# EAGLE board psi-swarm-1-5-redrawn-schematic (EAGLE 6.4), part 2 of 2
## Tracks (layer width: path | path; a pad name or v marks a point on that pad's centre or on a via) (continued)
N$38  (via drill 0.25 pad 0.65, 0.35 pad 0.75) (continued)
  Top 0.3: v24.6,17.68 23.1,17.68 22.55,18.23 22.55,20.08 22.45,20.18
  Top 0.305: U$16.P$2 79.9,19.58 78,17.68 76.6,17.68 73.7,14.78 62.3,14.78 v62.2,14.68 | 22.45,20.18 22.45,21.63 21.9,22.18 19.6,22.18 v19.5,22.28 | v15.05,22.38 U$17.3
  Bottom 0.305: v62.2,14.68 62.2,11.58 61.2,10.58 57.5,10.58 55.6,8.68 46.7,8.68 45,10.28 42.05,10.28 41.45,9.68 36.1,9.68 35.5,10.28 34.95,10.78 35,16.28 34.4,16.88 28.9,16.88 27.7,18.08 24.7,18.08 24.6,17.98 v24.6,17.68 | v19.5,22.28 15.15,22.28 v15.05,22.38
N$39  (via drill 0.25 pad 0.6)
  Top 0.2: IR3.CATHODE 99.46,32.29 98.97,32.78 | 98.97,32.78 N2.3 | v97.5,28.28 96.8,28.28 96.8,32.78 98.97,32.78 | v32,6.98 33,7.88 37.8,6.18 36.6,3.58 39.6,2.58 46.4,1.28 48,1.58 v48,1.88
  Top 0.254: IR5.CATHODE 30.7,7.28 v31.7,9.88 | v11.1,24.28 11,24.28 11,24.78 8,24.78 5.1,29.48 7.1,30.38 7.1,30.58 5.6,33.88 5.2,33.98 3.1,33.18 IR6.CATHODE
  Bottom 0.2: IR4.CATHODE 70.49,5.78 69.7,6.58 | 69.7,6.58 69.5,7.08 | 74.6,9.08 75.5,6.68 80.2,9.18 85.8,13.38 91.3,19.18 v97.5,28.28 | IR5.CATHODE 31.3,5.38 v32,6.98 | v48,1.88 48,1.58 55.7,1.58 61.8,2.48 67.9,4.18 67.4,5.58 69.7,6.58
  Bottom 0.254: v31.7,9.88 31.6,9.68 27.7,11.38 27.2,11.18 27.1,11.08 26.4,9.78 22.8,11.78 19.5,14.58 18.95,15.13 18.95,15.78 18.45,16.28 17.5,16.28 14.3,19.48 14.3,20.28 13.9,20.78 13.2,20.78 12.9,20.38 11,22.38 11,24.18 v11.1,24.28 | 74.6,9.08 73.8,8.78 73.6,9.28 73.1,9.48 72.4,9.18 72.2,8.38 69.5,7.08
N$40  (via drill 0.25 pad 0.6)
  Top 0.254: v54.7,98.88 RA3.1A
  Bottom 0.2: 31.8,99.08 33.2,99.08 33.9,99.78 37,100.88 37.5,100.88 38.1,101.08
  Bottom 0.25: 38.1,101.08 38.1,101.58 38.5,101.98
  Bottom 0.254: 27.8,98.88 27.8,99.06 IR_B1.P1-ANODE 29.3,98.78 31.3,99.58 31.8,99.08 | 38.5,101.98 41.9,102.78 41.9,103.18 43.2,103.48 44.5,102.18 49.7,102.18 52.3,99.58 54.7,99.58 v54.7,98.88
N$41  (via drill 0.25 pad 0.65)
  Top 0.2: U$15.3 19.66,28.23 U$15.8 | v28.7,66.48 31.2,68.98 34.5,68.98 v34.8,69.28 | v34.8,84.18 34.8,85.63 R26.2 | 22.25,29.78 22.25,28.3 U$4.10
  Top 0.254: C1.1 22.1,30.28 22,30.18 | 20.43,28.28 U$15.3
  Top 0.305: 22.14,28.04 22,28.18
  Top 0.6: 20.43,28.28 20.43,28.3 20.55,28.43 21.75,28.43 | 21.75,28.43 22,28.18 | 22,30.18 22,28.68 21.75,28.43 | 22.14,28.04 22.14,29.67 22.25,29.78
  Top 0.61: U$2.+ 22.95,39.71 22.95,31.73 22.6,31.38 C1.1
  Bottom 0.2: U$2.+ 24.04,43.44 21.2,46.28 21.2,47.08 21,47.28 21,47.98 21.4,48.38 21.4,55.68 25.8,60.08 27.6,60.08 28.8,61.28 28.8,66.38 v28.7,66.48 | v34.8,69.28 v34.8,84.18
N$42
  Top 0.2: U$4.9 22.99,29.07 23,29.08 23.5,29.08 23.7,29.28 23.7,36.78 25.6,38.68 29.3,38.68 30.2,37.68 35.65,37.68 TH1.2
N$43
  Top 0.61: HB_L.P$1 37.7,55.48 32.1,55.48 32.1,58.48 LEFT_MOTOR.MOTOR+
N$44
  Top 0.61: LEFT_MOTOR.MOTOR- 32,53.18 36.4,53.18 36.4,51.22 HB_L.P$7
N$46  (via drill 0.25 pad 0.6)
  Top 0.254: v49.1,100.28 49,100.18 47.74,100.18 RA1.3A
  Bottom 0.254: IR1.ANODE 72.6,100.38 58.6,100.38 57.9,99.68 55.9,99.68 55.5,99.28 55.5,98.68 55.1,98.18 51.3,98.18 v49.1,100.28
N$47  (via drill 0.25 pad 0.6)
  Top 0.2: RA1.4A 47.1,98.28 47.1,97.18 47.3,96.98 v47.8,96.98
  Top 0.254: v96.15,78.53 96.3,78.38 99,71.58 IR2.ANODE
  Bottom 0.2: 88.1,89.28 88.1,87.68 87.55,87.13 87.55,86.63 87.8,86.33 88.75,86.33 90.1,87.68 94.14,82.87 | v47.8,96.98 49,96.98 49.5,96.48 54,96.48 55.8,94.68 59.8,94.68 60.9,95.78 61.1,95.78
  Bottom 0.254: 61.1,95.78 81.5,95.78 81.6,95.68 83.9,93.53 84.55,93.53 85.4,92.78 85.4,91.98 88.1,89.28 | 93.9,83.18 94.14,82.87 95,81.78 96.4,78.93 v96.15,78.53
N$48  (via drill 0.25 pad 0.6, 0.25 pad 0.65)
  Top 0.2: v67.6,31.78 67.4,31.98 55.4,31.98 55,32.38 34.4,32.38 v34.1,32.08 | v11.9,29.38 RA2.1A
  Bottom 0.2: IR3.ANODE 92.87,31.11 92.45,31.58 91.5,31.58 90.4,30.48 89.6,30.48 88.85,31.13 82.85,31.13 82.2,31.78 80.95,31.78 80.5,31.38 73.2,31.38 72.8,30.98 71.5,30.98 71.1,31.38 68,31.38 v67.6,31.78 | v34.1,32.08 20.6,32.08 19.55,33.13 17.6,33.13 16.55,32.78 16.25,32.48 16.25,30.38 12,30.38 RA2.1A v11.9,29.38
N$49  (via drill 0.25 pad 0.65)
  Top 0.2: v13.15,29.38 13.15,30.26 RA2.2A
  Bottom 0.2: IR4.ANODE 68.94,4.42 68.1,3.58 62.2,1.98 54.8,0.98 46,1.08 39.3,2.28 34.9,3.68 36,6.48 27.8,10.08 27.7,9.98 26.9,8.18 21.8,11.08 15.9,15.88 10.5,22.08 10.5,24.58 11.8,25.88 11.8,26.48 12.4,27.08 12.85,27.08 13.6,27.83 13.6,28.93 v13.15,29.38
N$50  (via drill 0.25 pad 0.6)
  Top 0.2: RA2.3A 14.45,31.18 9.55,31.18 v9.35,30.98
  Bottom 0.254: IR5.ANODE 26.9,6.98 20.9,10.38 14.4,15.58 9.1,21.88 9.1,24.08 9.4,24.38 v9.35,30.98
N$51
  Top 0.2: RA2.4A 15.71,31.42 15.35,31.78 7.25,31.78 7,32.03 6.05,34.38 4.65,34.68 3.9,36.53 IR6.ANODE
N$52  (via drill 0.25 pad 0.6)
  Top 0.2: v9.1,75.38 8.9,75.48 9.6,77.08 9.7,78.18 9.1,79.78 8.9,79.98 10.1,82.08 11.4,82.08 12.1,82.68 12.1,84.18 11.9,84.38 11.9,85.58 12.4,86.28 23.8,86.28 24,86.48 25,86.48 25.3,86.78 25.3,92.78 v21.45,92.78 | RA1.1A 48.4,102.68 48.7,102.38 48.7,100.98 48.5,100.78 43.5,100.78 42.9,100.18 41.7,100.18 41.3,99.78 41.3,97.58 40.2,96.48 37.5,96.48 37,95.98 32.25,95.98 31.82,96.41 31.4,96.68 31.4,96.98 27.7,96.98 25.8,96.08 v25.8,95.08
  Bottom 0.2: IR7.ANODE v9.1,75.38 | v21.45,92.78 21.6,92.78 21.8,92.98 24.15,92.98 25.1,93.93 25.1,94.58 v25.8,95.08
N$53
  Top 0.254: RA1.2A 46.3,101.41 46.27,101.38 45.6,101.38 45.5,101.48 45.5,102.48 46.3,103.28 46.3,107.08 40.4,106.18 IR8.ANODE
N$54  (via drill 0.25 pad 0.6)
  Top 0.254: 38.3,100.68 34.3,100.68 33,101.98 | 33,101.98 33,102.76 IR8.CATHODE | N1.3 40.27,98.71 38.3,100.68 | 38.3,100.68 42.8,100.68 v45.6,103.48 | v97.85,72.38 v96.3,72.38 | v78.4,94.98 78.4,95.28 77.3,96.38 75.8,97.78 74.5,97.78 74.2,97.48 70.6,97.48 70.6,99.68 69.7,100.08 v64,102.28 | 33,101.98 32.9,101.98 31.3,100.38 23.2,96.88 23.2,95.08 v23.5,95.08 | v14.6,87.08 14.5,87.08 14.1,86.68 12.2,86.68 11.5,85.78 11.5,84.18 11.7,83.98 11.7,82.98 11.3,82.58 9.9,82.58 8.1,79.78 8.6,79.58 9.2,78.18 9.1,77.18 8.1,74.48 v8.4,74.48
  Bottom 0.2: 87.6,85.88 88.9,85.88 90.1,87.08 94.5,81.48
  Bottom 0.254: v45.6,103.48 50.1,103.48 52.9,100.68 56.6,100.68 56.9,100.98 57.2,101.38 58.1,101.38 58.6,100.88 | 58.6,100.88 71.44,100.88 IR1.CATHODE | IR2.CATHODE v97.85,72.38 | v96.3,72.38 95.5,77.28 95,77.28 95,80.48 94.5,81.48 | v78.4,94.98 78.4,95.18 81.4,95.18 83.65,93.08 84.35,93.08 84.9,92.58 84.95,92.53 84.95,91.83 87.65,89.13 87.65,87.88 87.1,87.33 87.1,86.48 87.6,85.88 | v64,102.28 63.5,102.28 63.5,101.88 60.1,101.88 59.9,102.18 58.9,102.18 58.6,101.78 58.6,100.88 | v23.5,95.08 23.5,94.18 23.3,93.98 19.9,93.98 14.1,87.98 14.1,87.08 v14.6,87.08 | v8.4,74.48 IR7.CATHODE
N$55  (via drill 0.25 pad 0.6)
  Top 0.254: v57.7,100.68 57.2,100.18 55.9,100.18 RA3.2A
  Bottom 0.254: IR_B2.P1-ANODE 44.9,104.54 44.9,102.88 45.3,102.78 49.9,102.78 52.5,100.18 57.2,100.18 v57.7,100.68
N$56  (via drill 0.25 pad 0.6)
  Top 0.254: v54.7,101.38 55.9,101.38 RA3.3A
  Bottom 0.254: IR_B3.P1-ANODE 54.7,105.18 v54.7,101.38
N$57  (via drill 0.25 pad 0.6)
  Top 0.254: RA3.4A v57.5,102.69 v57.5,102.68
  Bottom 0.254: v57.5,102.68 62.26,102.68 IR_B4.P1-ANODE
N$58  (via drill 0.25 pad 0.6)
  Top 0.254: v55.9,97.08 54.95,97.08 R15.1
  Bottom 0.254: IR_B5.P1-ANODE 77.65,97.23 77,96.58 68.6,96.58 68.3,96.88 68.3,97.68 68.5,97.88 68.5,98.58 68.3,98.78 61.8,98.78 | 59.1,96.08 56.9,96.08 v55.9,97.08
  Bottom 0.256: 59.1,96.08 59.75,96.73 59.9,97.03 59.9,98.18 60.1,98.58 60.35,98.78 61.8,98.78
N$59  (via drill 0.25 pad 0.6)
  Top 0.254: v64.3,104.08 64.4,104.08 66.7,101.78 73.8,98.88 v73.8,98.18 73.8,98.28 N3.3
  Bottom 0.2: 63.3,104.58 61.5,104.88 60.4,104.28 IR_B4.P2-CATHODE 57.3,104.98 56.7,104.98 55.5,106.58 55.1,106.58 54.5,105.98 51.5,105.98 50.7,105.18 IR_B3.P2-CATHODE 46.8,105.18 46.3,105.68 45.4,105.68 43.7,105.28 43.4,104.38 IR_B2.P2-CATHODE
  Bottom 0.254: 63.3,104.58 63.8,104.58 v64.3,104.08 | v73.8,98.18 IR_B5.P2-CATHODE | IR_B1.P2-CATHODE 26.7,98.58 26.3,99.28 27.8,100.08 28.2,100.08 28.7,99.48 29.1,99.38 29.4,99.38 36.7,102.18 36.4,102.78 IR_B2.P2-CATHODE
N$60  (via drill 0.25 pad 0.6)
  Top 0.2: v66.8,22.48 63.63,22.48 U1.7
  Bottom 0.2: SW1.P1 80.9,29.28 66.8,29.33 v66.8,22.48
N$61
  Top 0.2: SW1.P3 77.4,19.28 66.5,19.28 64.6,21.18 U1.8
N$62
  Top 0.2: SW1.P2 81.65,25.63 79.55,23.48 77.3,23.48 76.7,22.88 76.7,20.98 76.3,20.58 66,20.58 64.8,21.78 62.4,21.78 62.2,21.58 62.2,20.18 62.5,19.88 63.6,19.88 U1.9
N$63
  Top 0.2: SW1.P5 87.7,26.63 83.3,21.98 81.45,21.98 77.7,18.18 75.4,18.18 75.2,17.98 65.1,17.98 64.5,18.58 63.68,18.58 U1.10
N$64  (via drill 0.25 pad 0.6)
  Top 0.2: v61.9,17.38 U1.11
  Bottom 0.2: SW1.P6 91.1,29.53 83,29.48 82.2,28.68 80.9,28.68 80.7,28.88 67.4,28.88 67.4,15.38 61.7,15.38 61.7,17.38 v61.9,17.38
N$65
  Top 0.254: U2.21 51.62,26.25 R2.1
N$67
  Top 0.254: RA4.9 39.3,17.39 U2.11
N$68
  Top 0.254: U2.10 37.12,18.63 RA4.10
N$69
  Top 0.254: U2.9 37.12,19.9 RA4.11
N$70
  Top 0.254: U2.8 37.12,21.17 RA4.12
N$71
  Top 0.254: U2.7 37.12,22.44 RA4.13
N$72
  Top 0.254: U2.6 37.12,23.71 RA4.14
N$73
  Top 0.254: U2.5 39.1,24.98 37.12,24.98 RA4.15
N$74
  Top 0.254: U2.4 37.12,26.25 RA4.16
N$75
  Top 0.254: U2.20 50.99,24.98 RA5.9
N$76
  Top 0.254: RA5.10 48.69,23.7 U2.19
N$77
  Top 0.254: U2.18 50.99,22.44 RA5.11
N$78
  Top 0.254: RA5.12 48.69,21.16 U2.17
N$79
  Top 0.254: U2.16 50.99,19.9 RA5.13
N$80
  Top 0.254: RA5.14 48.69,18.62 U2.15
N$81
  Top 0.254: U2.14 50.99,17.36 RA5.15
N$82
  Top 0.254: RA5.16 48.69,16.08 U2.13
N$83
  Top 0.2: U1.20 74.41,24.98 75.8,26.38 75.8,28.29 SW2.1
N$84
  Top 0.2: SW2.2 85.63,35.11 84.7,34.18 82.3,34.18 76.2,28.08 76.2,26.18 74.3,24.28 73.54,24.28 U1.19
N$85
  Top 0.2: SW2.3 87.8,35.58 86,33.78 82.5,33.78 76.6,27.88 76.6,25.98 74.4,23.78 74.4,23.38 74.1,23.08 73.61,23.08 U1.18
N$86
  Top 0.2: SW2.4 90.6,35.58 88.4,33.38 82.7,33.38 77,27.68 77,25.78 74.8,23.58 74.8,23.08 74.3,22.58 74.3,21.98 74.1,21.78 73.58,21.78 U1.17
N$87  (via drill 0.25 pad 0.6)
  Top 0.2: LED1.P2-CRED 51.5,105.58 51.9,105.18 55.6,105.18 56,105.58 56,107.28 58.3,106.98 64.1,105.88 67.4,102.58 75,99.38 75.6,99.38 84.7,90.28 84.7,89.68 84.3,89.28 84.3,87.88 85.3,86.88 86.7,86.88 88,88.18 88.4,88.18 89.65,86.93 91.5,86.93 93.5,84.93 93.5,78.33 94.85,76.98 94.85,68.88 93.5,67.53 93.5,50.08 93.3,49.88 80.9,49.88 v80.7,50.08 | RA4.1 30.11,33.59 31.3,34.78 56.2,34.78 56.6,34.38 66.2,34.38 67.1,35.28 67.5,35.28 v67.7,35.48
  Bottom 0.2: v67.7,35.48 68.8,35.48 69.9,34.38 74.7,34.38 74.7,49.28 76.8,51.38 79.6,51.38 80.7,50.28 v80.7,50.08
N$88  (via drill 0.25 pad 0.6)
  Top 0.2: LED1.P3-CGREEN 50.9,104.78 55.8,104.78 56.5,105.48 56.5,106.78 58.2,106.58 63.8,105.48 64.4,104.78 67.1,102.08 74.8,98.98 75.4,98.98 84.2,90.18 84.2,89.78 83.8,89.38 83.8,87.78 85.1,86.48 86.9,86.48 88,87.58 88.4,87.58 89.45,86.53 91.35,86.53 93.1,84.78 93.1,78.03 94.45,76.68 94.45,68.98 93.1,67.63 93.1,50.38 93,50.28 81.4,50.28 81,50.68 80.4,50.68 80.2,50.48 v79.6,50.48 | RA4.2 30.83,25.01 31.4,25.58 31.4,33.68 32.1,34.38 56,34.38 56.4,33.98 66.6,33.98 67.1,34.48 67.1,34.68 67.3,34.88 v68.3,34.88
  Bottom 0.2: v68.3,34.88 68.8,34.88 69.7,33.98 75.1,33.98 75.1,49.08 76.9,50.88 79.2,50.88 v79.6,50.48
N$90  (via drill 0.25 pad 0.6)
  Top 0.2: LED2.P2-CRED 87.95,89.73 88,89.73 88,89.68 89.95,87.73 91.85,87.73 94.3,85.28 94.3,79.08 95.65,77.73 95.65,68.33 94.3,66.98 94.3,49.18 94.2,49.08 79.6,49.08 v79.4,49.28 | RA4.3 30.86,23.74 32,24.88 32,33.48 32.5,33.98 55.8,33.98 56.2,33.58 66.8,33.58 67.5,34.28 v67.7,34.28
  Bottom 0.2: v67.7,34.28 68.5,34.28 68.9,34.08 69.5,33.58 75.4,33.58 75.5,33.68 75.5,48.78 77.2,50.48 78.7,50.48 79.4,49.48 v79.4,49.28
N$91  (via drill 0.25 pad 0.6)
  Top 0.2: LED2.P3-CGREEN 86.25,92.23 85.6,91.58 85.6,91.48 85.65,91.48 89.8,87.33 91.65,87.33 93.9,85.08 93.9,78.68 95.25,77.33 95.25,68.48 93.95,67.18 93.95,49.63 93.8,49.48 80.3,49.48 79.9,49.88 v78.4,49.88 | RA4.4 31.59,22.47 32.4,23.28 32.4,33.18 32.8,33.58 55.6,33.58 56,33.18 67,33.18 67.6,33.68 v68.3,33.68
  Bottom 0.2: v68.3,33.68 68.7,33.68 69.3,33.18 75.6,33.18 75.9,33.48 75.9,48.58 77.1,49.78 78.4,49.78 v78.4,49.88
N$92  (via drill 0.25 pad 0.6)
  Top 0.2: RA4.5 31.72,21.2 32.8,22.28 32.8,32.98 33,33.18 55.4,33.18 55.8,32.78 67.5,32.78 v67.7,32.98 | v78.5,48.08 78.7,48.28 94.8,48.28 95.1,48.58 95.1,62.63 LED3.P2-CRED
  Bottom 0.2: v67.7,32.98 68.7,32.98 68.9,32.78 75.8,32.78 76.3,33.28 76.3,48.28 77.3,49.28 77.9,49.28 78.5,48.68 v78.5,48.08
N$93  (via drill 0.25 pad 0.6)
  Top 0.2: RA4.6 31.35,19.93 33.2,21.78 33.2,32.68 33.3,32.78 55.2,32.78 55.6,32.38 v68.2,32.38 | v77.6,48.68 94.5,48.68 94.7,48.88 94.7,64.23 95.25,64.78 96.15,64.78 LED3.P3-CGREEN
  Bottom 0.2: v68.2,32.38 76.1,32.38 76.7,32.98 76.7,47.78 v77.6,48.68
N$94
  Top 0.2: RA4.7 30.19,18.58 32.1,18.58 32.4,18.28 32.4,14.78 32.8,14.38 52.2,14.38 53.9,16.08 53.9,17.58 56.8,20.48 59.2,20.48 59.8,19.88 59.8,14.18 60.4,13.58 77.4,13.58 77.65,13.33 80.05,13.33 81.6,14.88 84.6,14.88 87.1,17.38 87.7,17.38 LED4.P2-CRED
N$95  (via drill 0.25 pad 0.6)
  Top 0.2: LED4.P3-CGREEN 88.87,18.41 88.4,18.88 88,18.88 84.5,15.38 81.5,15.38 79.85,13.73 77.9,13.73 77.65,13.98 60.6,13.98 60.2,14.38 60.2,14.78 v60.5,15.08 | v53.1,16.38 53.1,15.98 51.9,14.78 33.1,14.78 32.9,14.98 32.9,18.48 32.1,19.28 28.9,19.28 28.7,19.08 28.7,17.48 28.8,17.38 30.1,17.38 RA4.8
  Bottom 0.2: v60.5,15.08 60.5,14.98 53.5,14.98 53.5,16.38 v53.1,16.38
N$96
  Top 0.2: LED5.P2-CRED 51.5,4.08 57.9,10.68 57.9,15.99 RA5.1
N$97
  Top 0.2: LED5.P3-CGREEN 53.25,5.23 58.3,10.48 58.3,15.18 58.5,15.38 59.2,15.38 59.3,15.48 59.3,17.08 59,17.38 58.02,17.38 RA5.2
N$98
  Top 0.2: RA5.3 57.95,18.58 55.7,18.58 54.4,17.28 54.4,15.88 52.5,13.98 32.7,13.88 32.6,13.88 32,14.48 28.5,14.48 27.4,15.58 19.8,15.58 18.75,16.63 16.9,16.63 15.45,18.08 15.45,18.03 LED6.P2-CRED
N$99
  Top 0.2: 16.1,15.98 LED6.P3-CGREEN 16.07,16.18 18.55,16.18 18.85,15.88 18.85,15.38 19.2,15.03 19.85,15.03 24.9,14.98 25.1,15.18 27.1,15.18 28.3,13.98 31.8,13.98 32.2,13.58 32.2,13.48 52.7,13.48 54.9,15.68 54.9,17.08 55.8,17.98 59.2,17.98 59.4,18.18 59.4,19.38 58.8,19.98 58.08,19.98 RA5.4
N$100  (via drill 0.25 pad 0.6)
  Top 0.2: v27.3,48.18 26.6,48.88 7.15,48.88 6.6,49.43 6.6,60.03 6.85,60.28 7.8,60.28 7.85,60.33 7.85,62.68 LED7.P2-CRED | RA5.5 56.62,21.16 56.1,21.68 56.1,25.98 56.7,26.58 v56.7,26.78 | v28.1,35.08 28.1,33.98 28.6,33.48 29.4,33.48 31.1,35.18 56.6,35.18 v56.9,34.98
  Bottom 0.2: v27.3,48.18 27.3,47.98 27.7,47.58 27.7,35.48 v28.1,35.08 | v56.9,34.98 56.9,26.98 v56.7,26.78
N$101  (via drill 0.25 pad 0.6)
  Top 0.2: v21.7,47.68 21,48.38 6.85,48.38 6.2,49.03 6.2,60.73 LED7.P3-CGREEN | RA5.6 57.05,22.43 56.6,22.88 56.6,25.58 56.9,25.88 v57.4,25.88 | v29.1,34.18 29.4,34.18 30.8,35.58 57.4,35.58 v57.8,35.28
  Bottom 0.2: v21.7,47.68 21.7,46.48 23.2,44.98 25.3,44.98 25.6,45.28 25.6,46.18 26,46.53 26.9,46.53 27.15,46.23 27.2,34.88 27.9,34.18 v29.1,34.18 | v57.8,35.28 57.8,26.28 v57.4,25.88
N$102  (via drill 0.25 pad 0.6)
  Top 0.2: LED8.P2-CRED 15,89.98 15,89.88 13.5,88.38 13.2,88.38 12.6,88.98 12.4,88.98 11.4,87.88 10.8,87.18 9.9,86.08 9,84.88 7.4,82.58 6.9,81.78 5.2,78.68 6.9,78.08 7.1,77.98 7.2,77.88 7.3,77.68 7.3,77.58 5.1,71.98 6.1,71.98 6.9,71.18 6.9,68.38 7,68.28 7.9,68.28 8.3,67.88 8.3,64.58 8.7,64.18 8.7,59.88 8.25,59.43 7.55,59.43 7.4,59.28 7.4,50.08 7.6,49.88 v28.5,49.88 | v29.1,35.98 29.5,36.38 58.65,36.38 59.3,35.73 v59.3,35.08 | RA5.7 59.12,23.7 v59.4,23.98
  Bottom 0.2: v28.5,49.88 28.6,49.88 29.1,49.38 29.1,48.48 28.5,47.98 28.5,36.48 v29.1,35.98 | v59.3,35.08 v59.4,23.98
N$103  (via drill 0.25 pad 0.6)
  Top 0.2: LED8.P3-CGREEN 12.4,89.68 10.5,87.48 9.4,86.08 8.1,84.28 6.6,82.08 4.6,78.48 6.7,77.68 6.8,77.58 6.8,77.48 4.5,71.68 4.5,71.58 5.9,71.58 6.5,70.98 6.5,67.98 6.6,67.88 7.7,67.88 7.9,67.68 7.9,64.28 8.3,63.88 8.3,60.08 8.1,59.88 7.45,59.88 7,59.43 7,49.63 7.2,49.43 27.3,49.43 27.85,48.88 28.1,48.88 v28.2,48.98 | v29.1,35.08 30,35.98 58.2,35.98 v58.5,35.68 | v58.5,25.98 58.5,25.48 RA5.8
  Bottom 0.2: v28.2,48.98 28.2,48.28 28.1,48.18 28.1,35.98 v29.1,35.08 | v58.5,35.68 v58.5,25.98
N$104
  Top 0.61: RIGHT_MOTOR.MOTOR- 69.11,58.48 HB_R.P$1
N$105
  Top 0.254: HB_R.P$6 66.6,51.22 66.6,50.18 64.3,50.18 64.3,54.18
  Top 0.61: HB_R.P$2 HB_R.P$3 | HB_R.P$3 C6.1 | VR_R.4 62,50.88 62,54.18 64.3,54.18 66.56,54.18 HB_R.P$3
N$107
  Top 0.61: HB_R.P$7 67.9,51.22 68.2,49.68 RIGHT_MOTOR.MOTOR+
N$108
  Top 0.2: 35.2,51.22 35.2,50.08 37.1,50.08 37.1,54.78 39,54.78 39,55.08
  Top 0.305: HB_L.P$6 35.2,51.22
  Top 0.61: 35.95,58.28 35.95,56.94 HB_L.P$2 HB_L.P$3 | 35.95,58.28 C2.1 | VR_L.4 43.6,50.88 43.6,55.08 39,55.08 38.9,55.08 38.9,58.28 35.95,58.28
N$109  (via drill 0.35 pad 0.75)
  Top 0.305: U4.3 U4.4
  Top 0.61: U4.4 67.52,83.15 | v83.9,72.63 84.2,72.3
  Top 0.8: 67.52,83.15 v67.05,83.13 | v73.95,81.28 73.95,78.63 v74.65,77.93 | 84.2,72.3 L2.1
  Bottom 0.8: v67.05,83.13 67.95,82.28 72.95,82.28 v73.95,81.28 | v74.65,77.93 80.35,77.93 83.75,74.53 83.75,72.63 v83.9,72.63
PGDIR  (via drill 0.25 pad 0.6)
  Top 0.254: v60.9,42.48 60.8,42.48 60.8,42.28 40,42.28 39.4,42.88 31.3,42.88 30.7,42.28 19.45,42.28 17.65,40.43 VR_IR.5 | v61.9,23.68 61.9,23.71 U1.6
  Bottom 0.254: v60.9,42.48 60.9,31.78 59.9,30.78 59.9,29.38 60.9,28.38 60.9,23.68 v61.9,23.68
PGDL  (via drill 0.25 pad 0.6)
  Top 0.254: VR_L.5 44.84,44.08 57.4,44.08 v57.4,44.38 | v62,26.18 62,26.25 U1.4
  Bottom 0.254: v57.4,44.38 57.4,44.08 57.6,44.08 57.8,43.88 61.5,43.88 61.6,43.78 61.5,31.58 60.5,30.58 60.5,29.58 61.6,28.48 61.6,26.18 v62,26.18
PGDR  (via drill 0.25 pad 0.6)
  Top 0.254: VR_R.5 63.24,49.28 v63.7,49.28 | v65.4,24.98 U1.5
  Bottom 0.254: v63.7,49.28 63.7,31.48 65.4,31.48 v65.4,24.98
PIC_CO_1  (via drill 0.25 pad 0.65)
  Top 0.2: U$7.P$8 85.38,84.25 86.05,83.68 v86.45,83.68 | v91.3,53.08 v91.3,51.58 | v89.7,42.48 86.55,42.48 78.8,34.73 v78.8,34.38 | U1.16 76.42,19.9 v78.4,21.88 | v84.95,31.83 v84.95,28.43
  Bottom 0.2: v86.45,83.68 88.85,81.18 88.85,80.28 92.35,76.78 92.35,58.63 93.1,57.88 93.1,56.43 93.35,56.18 94.9,56.18 95.15,55.93 95.15,54.23 94.65,53.73 91.35,53.73 91.3,53.68 v91.3,53.08 | v91.3,51.58 91.3,46.33 91,46.03 89.95,46.03 89.7,45.78 v89.7,42.48 | v78.4,21.88 78.4,22.33 81.3,25.23 82.3,25.23 84.95,27.88 v84.95,28.43 | v78.8,34.38 78.8,34.33 79.05,34.08 79.8,34.08 81.65,32.23 84.9,32.23 84.95,32.18 v84.95,31.83
PIC_CO_2  (via drill 0.25 pad 0.65)
  Top 0.2: 85.12,79.1 U$7.P$7 85.12,77.71 85.25,77.58 86.2,77.58 86.4,77.38 88.7,77.38 88.9,77.58 v89.1,77.58 | v88.9,53.33 v88.9,51.43 | v88.85,40.18 88.85,39.88 91.65,37.08 91.65,34.43 91.15,33.93 89.6,33.93 88.55,32.88 84.45,32.88 83.2,31.63 83.2,23.33 82.45,22.58 81.35,22.58 77.5,18.73 73.07,18.73 U1.15
  Bottom 0.2: v89.1,77.58 89.05,77.38 90.15,76.28 90.15,69.13 91.55,67.73 91.55,57.68 91.25,57.38 90.15,57.38 89.95,57.18 89.95,54.38 v88.9,53.33 | v88.9,51.43 88.9,40.23 v88.85,40.18
PIC_ICSPCLK  (via drill 0.25 pad 0.65)
  Top 0.2: PIC.3 40.86,5.74 | 40.86,5.74 40.3,5.18 40.3,4.15 U$19.2 | U$4.7 24.01,28.89 24.3,29.18 24.3,36.68 25.4,37.88 v29.2,37.88 | v36.4,64.08 46.5,64.08 46.5,70.18 48,71.68 50.3,71.68 51.7,73.08 51.7,73.63 52,73.93 53,73.93 53.35,74.28 v55.25,74.28 | U5.14 62.3,77.18 61.5,76.38 61.5,74.98 60.8,74.28 v58.1,74.28 | 40.86,5.74 40.76,5.74 40.3,5.28 40.3,3.18 40.5,2.98 46.4,1.68 47.3,1.98 47.3,3.28 47.6,3.58 50.6,3.58 v50.7,3.68 | v53.8,7.78 54.4,7.78 57.3,10.68 57.3,14.68 56.5,15.48 56.5,16.88 v56.1,17.28 | v48.9,45.78 47.5,47.08 v45.8,47.08 | v43.7,47.98 43.7,45.18 43,44.88 41.5,44.88 v40.6,45.98
  Bottom 0.2: v29.2,37.88 29.1,37.98 29.1,38.18 28.9,38.38 28.9,45.98 30.6,47.68 35.1,47.68 35.95,48.53 | 35.95,48.53 36.3,48.88 36.3,63.98 v36.4,64.08 | v50.7,3.68 53.4,6.38 53.4,7.38 v53.8,7.78 | v56.1,17.28 56.1,30.48 54.4,32.18 49.1,32.18 48.6,32.68 48.6,45.78 v48.9,45.78 | v45.8,47.08 44.6,47.08 v43.7,47.98 | v40.6,45.98 39.1,45.98 35.95,48.53 | v55.25,74.28 v58.1,74.28
PIC_ICSPDAT
  Top 0.2: PIC.1 49.16,7.62 49.3,7.48 49.3,5.28 49,4.98 45.9,4.98 45.6,5.28 42.9,5.28 42.4,4.78 42.4,3.83 U$19.3
PIC_VPP  (via drill 0.25 pad 0.65)
  Top 0.2: PIC.6 49.94,7.62 49.8,7.48 49.8,4.98 49.4,4.58 44.8,4.58 44.3,4.08 44.3,3.31 U$19.4 | SW3.1 25.9,11.28 v25.9,14.58 | v25.9,16.68 26.5,16.68 26.7,16.48 31.35,16.48 31.6,16.73 31.6,17.78 v31.7,17.78 | v41.7,11.78 41.7,11.48 41.8,11.38 41.8,8.38 v42.1,8.38
  Bottom 0.2: v25.9,14.58 v25.9,16.68 | v31.7,17.78 34.5,17.78 34.5,17.58 40.3,11.78 v41.7,11.78 | U$19.4 44.5,3.51 44.5,5.48 43.3,5.48 42.1,6.68 v42.1,8.38
PIEZO  (via drill 0.25 pad 0.65)
  Top 0.2: N6.1 72.88,95.3 73.1,95.08 v74,95.08
  Top 0.254: U$7.P$11 v81.31,85.32 v81.3,85.33
  Bottom 0.2: v81.3,85.33 80.35,86.28 78.75,86.28 78.4,86.63 78.4,91.38 78.65,91.63 78.65,93.03 78.1,93.58 75.4,93.58 74.05,94.93 v74,95.08
RIGHTF  (via drill 0.25 pad 0.6)
  Top 0.254: U$1.P$63 32.5,62.83 32.5,60.98 62.35,60.98 v62.35,60.58 | 65.3,56.88 HB_R.P$4 65.3,57.08 v63.6,57.08
  Bottom 0.254: v62.35,60.58 62.4,57.68 63,57.08 v63.6,57.08
  Bottom 0.406: U$1.P$23 U$1.P$63
RIGHTR
  Top 0.254: U$1.P$64 35.1,62.83 35.1,61.48 62.55,61.48 | 72.3,60.58 72.3,55.48 71.5,54.78 67.8,54.78 67.4,54.38 67.4,53.88 66.9,53.38 65.3,53.38 HB_R.P$5 | 62.6,61.48 62.6,61.43 63.25,60.78 72.1,60.78
  Top 0.256: 62.55,61.48 62.6,61.48 | 72.1,60.78 72.3,60.58
  Bottom 0.406: U$1.P$24 U$1.P$64
SCL  (via drill 0.25 pad 0.6, 0.25 pad 0.65)
  Top 0.2: v24.2,85.88 13.2,85.88 12.5,85.18 12.5,82.38 12.2,82.08 12.2,80.21 ADC1.19 | U2.22 50.55,27.52 v50.7,27.68 51.1,28.08 54,28.08 55.4,29.48 61.3,29.48 61.7,29.08 62.1,29.08 62.5,29.48 65.7,29.48 67.66,27.52 U1.22 | 52.8,88.19 U$1.P$10 | v49,68.18 51,70.18 51,71.38 51.45,71.83 v55.3,71.83 | U$5.P$1 79.7,92.68 79.55,92.83 | v65.1,93.28 65.3,93.48 70.2,93.48 71.25,92.43 75.85,92.43 76.9,93.48 78.9,93.48 79.25,93.13 79.55,92.83 | v82.3,87.18 82.1,86.98 82.1,86.18 82.58,85.7 U$7.P$10 82.58,82.66 82.3,82.38 78.8,82.38 78.15,81.73 78.15,73.08 78.9,72.08 78.9,67.88 v79.15,67.63 | v79.3,92.53 79.55,92.83 | v46.5,54.08 46.5,54.18 49.2,56.88 v49.8,56.88 | v78.9,63.83 79.1,63.63 80.65,63.63 80.8,63.78 U$20.2-SCL 80.8,65.38 80.9,65.48 81.75,65.48 82.1,65.13 82.1,63.98 81.85,63.73 81.85,62.53 81.92,62.46 U$23.2 | v62.85,83.38 v62.84,83.37 EEPROM.1 61.39,83.28 59.7,83.28 | R17.2 59.7,83.28 | 59.7,83.28 v59.7,83.03 | v55,82.28 52.4,82.28 v52.25,82.38
  Top 0.254: ADC2.19 12.21,67.96 11.9,68.28 11.2,68.28 10.8,68.68 10.8,72.48 10.9,72.48 v11.2,72.78 | v12.4,77.58 12.2,77.78 12.2,80.18 ADC1.19 | v49,64.08 v49,68.18 | v50.9,84.68 50.9,85.78 52.2,85.78 52.8,86.38 53.1,86.38 v53.3,86.18 | U5.3 59.6,69.66 59.6,69.98 59.7,69.98 v59.7,72.48 | U$1.P$50 52.84,91.64 52.3,92.18 48.8,92.18 48.3,92.68 48.3,93.66 U$9.3-SCL
  Bottom 0.2: v24.2,85.88 39.8,85.88 40.8,86.88 51.4,86.88 52.3,85.98 52.3,85.88 52.8,86.38 52.8,88.19 U$1.P$10 | v50.7,27.68 49.9,28.48 49.8,28.48 47.3,30.98 47.3,47.88 47.1,48.08 47.1,54.68 | v49,64.08 49,61.88 48.3,61.18 48.3,60.98 48,60.68 47.2,60.68 47,60.48 47,55.08 47.1,54.88 47.1,54.68 | v50.9,84.68 52.25,83.33 v52.25,82.38 | v65.1,93.28 65.1,92.58 64.3,91.78 64.3,84.83 v62.85,83.38 | v82.3,87.18 82.8,87.68 82.8,91.58 82.2,92.18 81.8,92.18 81.1,91.48 79.7,91.48 79.3,91.88 v79.3,92.53 | 47.1,54.68 v46.5,54.08 | v49.8,56.88 49.2,56.88 49,56.68 49,54.18 49.05,54.13 | v78.9,63.83 79.15,64.08 v79.15,67.63 | U$18.2-SCL 49.1,54.08 49.05,54.13 | 49.05,54.13 49.05,51.33 49.35,51.03 56.45,51.03 U$26.SCL | v55.3,71.83 59.05,71.83 v59.7,72.48 | v59.7,83.03 59,83.03 58.25,82.28 v55,82.28
  Bottom 0.254: v11.2,72.78 11.2,76.88 11.9,77.58 v12.4,77.58 | v49,68.18 36.6,68.18 36.6,84.88 40.2,84.88 41.4,86.08 49.9,86.08 50.7,85.28 50.7,84.88 v50.9,84.68 | v53.3,86.18 53,86.18 52.8,86.38
  Bottom 0.406: U$1.P$10 U$1.P$50
SCL2
  Top 0.2: 42.68,65.56 U$1.P$27 42.7,65.39 | U$28.SCL 53.57,75.61 51.6,77.58
  Top 0.254: 42.7,65.39 42.7,67.18 45.4,69.88 45.4,73.98 48.2,76.78 50.8,76.78 51.6,77.58 51.6,78.53 52.2,79.18 54.05,79.18 55.65,80.78 55.65,84.58 56.4,85.33 R14.1
  Bottom 0.2: U$3.7-SCL 54.73,10.2 54.1,9.58 46.7,9.58 45.8,10.48 45.8,43.48 43.9,43.48 43.2,44.18 43.2,45.78 41.1,47.88 41.1,51.28 45.8,55.68 45.8,58.28 45.35,58.28 45,58.63 45,59.58 44.38,60.2 42.68,60.2 U$1.P$67
  Bottom 0.406: U$1.P$27 U$1.P$67
SDA  (via drill 0.25 pad 0.6, 0.25 pad 0.65)
  Top 0.2: ADC1.18 12.9,84.98 13.27,85.35 13.27,85.38 23.3,85.38 v23.6,85.08 | U2.23 50.31,28.79 v50.6,29.08 | v51.6,64.08 51.6,67.98 | 51.6,67.98 51.6,68.08 v52.25,68.73 | U1.23 69.08,28.79 67.9,29.98 67.9,30.48 67.6,30.78 54.7,30.78 54.5,30.58 v54.5,30.18 | v51.1,59.68 v47.7,59.68 | U$5.P$16 80.25,92.08 | 80.25,92.08 80.25,92.93 79.2,93.98 76.75,93.98 75.6,92.83 71.55,92.83 70.4,93.98 64.8,93.98 64.3,93.48 63.9,93.48 v63.8,93.38 | v82.8,86.38 83.4,85.78 83.8,85.78 83.8,84.75 U$7.P$9 83.85,82.28 83.55,81.98 79.65,81.98 79.4,81.73 79.4,72.78 79.3,72.68 79.3,68.58 80.15,67.73 80.15,67.43 | v80.8,92.08 80.25,92.08 | 80.15,67.43 U$20.6-SDA | U5.4 61.03,68.41 60.4,67.88 51.7,67.88 51.6,67.98 | v55.5,92.93 55.5,90.89 U$1.P$49 | 80.15,67.43 80.25,67.33 82.1,67.33 83.02,66.41 U$23.1 | EEPROM.3 59.95,81.49 | 59.95,81.49 58.81,81.49 R16.2 | v59.85,82.03 59.85,81.59 59.95,81.49
  Top 0.254: ADC2.18 12.87,68.3 12.4,68.78 11.6,68.78 11.3,69.08 11.3,71.48 v11.7,71.88 | v13.4,77.58 13.4,77.68 12.9,78.18 12.9,80.17 ADC1.18
  Bottom 0.2: v23.6,85.08 24.3,85.08 24.7,85.48 40.1,85.48 41.1,86.48 51.1,86.48 52.1,85.48 53.45,85.48 | 53.45,85.48 53.8,85.48 53.8,85.53 53.9,85.63 53.9,86.75 U$1.P$9 55.4,88.21 | v50.6,29.08 51.2,29.68 51.2,30.38 | 51.2,30.38 51.2,30.88 53.8,30.88 v54.5,30.18 | v51.6,64.08 51.6,62.08 51.1,61.58 v51.1,59.68 51.4,59.38 51.4,57.98 51.9,57.48 53,57.48 54,56.48 54,53.68 53.75,53.43 53.65,53.43 U$18.6-SDA | v52.25,68.73 52.1,68.93 52.12,80.98 52.87,81.68 | 51.2,30.38 51.1,30.28 48.6,30.28 47.7,31.18 47.7,48.18 47.5,48.38 47.5,55.18 47.4,55.28 47.4,59.38 v47.7,59.68 | U$1.P$49 57.69,93.18 60.55,93.18 61.7,94.33 62.55,94.33 63.5,93.38 v63.8,93.38 | v82.8,86.38 82.8,86.68 83.2,87.08 83.2,89.78 83.5,90.08 83.5,91.48 82.1,92.88 81.7,92.88 v80.8,92.08 | U$9.2-SDA 45.74,94.02 46.85,95.13 54,95.13 55.5,93.63 v55.5,92.93 | 52.87,81.68 52.87,84.9 53.45,85.48 | 52.87,81.68 59.5,81.68 v59.85,82.03
  Bottom 0.254: v11.7,71.88 11.9,72.08 11.9,76.38 12.3,76.78 12.6,76.78 v13.4,77.58 | U$26.SDA 54,53.08 53.65,53.43
  Bottom 0.406: U$1.P$49 U$1.P$9
SDA2  (via drill 0.25 pad 0.65)
  Top 0.2: U$1.P$28 45.3,65.45 45.3,67.48 46.1,68.28 46.1,73.08 47.2,74.18 50.7,74.18 51.3,74.78 52.65,74.78 v52.75,74.68 | R13.1 61.35,85.33 v61.3,85.28
  Bottom 0.2: U$3.6-SDA 52.66,11.38 47.1,11.38 46.4,12.08 46.4,44.98 46,45.38 44.3,45.38 41.6,48.08 41.6,51.08 46.2,55.48 46.2,60.48 45.22,61.46 U$1.P$68 | v61.3,85.28 61.05,85.28 60.45,84.68 60.4,73.88 59.85,73.33 54.16,73.33 U$28.SDA 52.75,74.22 v52.75,74.68
  Bottom 0.406: U$1.P$28 U$1.P$68
V_BATT
  Top 0.2: U$1.P$16 36.95,88.23 35.7,86.98 33.1,86.98 32.9,86.78 32.9,85.93 R26.1 32.85,84.73 32.2,84.08 31.2,84.08 30.6,84.68 30.6,85.83 R27.1
  Bottom 0.406: U$1.P$56 U$1.P$16
V_CURRENT  (via drill 0.25 pad 0.6)
  Top 0.2: 10.26,27.62 U6.6 10.74,27.68 v11.6,27.73 | U$1.P$15 39.35,88.23 36.7,85.58 36.7,84.18 v35.8,83.28 | v36,70.08 36,68.08 34.4,68.08 33.8,67.48 v33.8,64.08 | v29.2,55.78 26.1,52.68 8.95,52.68 v8.25,51.98
  Bottom 0.2: v35.8,83.28 35.8,70.28 v36,70.08 | v33.8,64.08 33.8,61.88 32.3,60.38 31.2,60.38 28.9,58.08 28.9,56.08 v29.2,55.78 | 10,28.03 v11.6,27.73 | 7.1,31.98 6.75,32.33 6.75,35.53 6.9,35.68 6.9,51.38 7.5,51.98 v8.25,51.98
  Bottom 0.254: 10,28.03 10,31.33 9.35,31.98 7.1,31.98
  Bottom 0.406: U$1.P$55 U$1.P$15
V_DC  (via drill 0.25 pad 0.65)
  Top 0.2: 26.4,46.08 26.4,47.08 v26.6,47.28 | v31.2,66.48 33.2,68.48 35.5,68.48 35.5,69.58 34.8,70.28 34.4,70.28 v34,69.88 | v31.7,84.78 31.7,86.78 31.3,87.18 31.3,89.38 31.4,89.48 34.86,89.48 35.06,89.68 U$1.P$57
  Top 0.254: R28.1 19.45,24.53 18.6,25.38 16.7,25.38 16.2,25.88 16.2,27.13 R22.2 16.15,27.83 17,28.68 17,29.58 v18.1,30.48 | v20.9,31.28 21.6,31.98 v21.6,34.88 | v26.35,45.83 26.3,45.98 26.4,46.08
  Bottom 0.2: v26.6,47.28 26.6,48.98 28.3,50.68 28.3,58.28 31.2,61.18 v31.2,66.48 | v34,69.88 34,83.88 33.5,84.38 32.1,84.38 v31.7,84.78
  Bottom 0.254: v18.1,30.48 20.1,30.48 v20.9,31.28 | v21.6,34.88 22.2,34.88 25.7,38.38 25.7,44.68 26.15,45.08 26.35,45.28 v26.35,45.83
  Bottom 0.406: U$1.P$57 U$1.P$17
V_IR3.3  (via drill 0.25 pad 0.6, 0.25 pad 0.65)
  Top 0.2: R6.2 20.75,60.43 19.25,59.03 15.9,59.03 14.9,60.28 14.9,61.29 ADC2.6 | v50.8,68.48 51.45,69.23 51.55,69.33 52.6,69.33 52.85,69.08 52.85,68.43 52.95,68.33 56.9,68.33 57.2,68.63 57.2,69.64 U5.1 57.22,72.65 57.9,73.33 61.55,73.33 61.75,73.13 62.3,72.58 U5.5 U5.6 | v37.4,71.78 37.4,72.68 37.2,72.88 | 12.6,17.68 12.6,17.58 15.7,14.48 20.8,10.38 24.1,8.28 26.7,6.78 27.7,6.58 28.5,8.58 30.1,7.88 31.4,10.68 32.5,10.28 31.95,8.83 | 15.95,92.23 LED8.P1-ANODE 15,92.88 12,89.88 10.7,88.38 9.2,86.58 7.8,84.68 6.1,82.08 4.9,79.98 4,78.28 4.2,78.18 6.3,77.38 3.8,71.18 5.7,71.18 6.1,70.78 6.1,65.53 LED7.P1-ANODE | LED4.P1-ANODE 85.6,13.18 80.1,9.08 77.84,7.9 75.3,6.58 74.45,8.62 71.7,7.38 71.6,6.28 71.2,6.08 71,6.08 70.4,6.88 67.4,5.58 68.1,3.58 61.7,1.88 54.8,0.98 54.4,0.68 49.9,0.68 49.8,0.78 49.8,1.83 LED5.P1-ANODE 49.8,1.08 46.5,0.88 39.2,2.28 36,3.28 37.1,5.88 33.3,7.28 32,6.18 31.4,6.38 31.4,7.48 31.95,8.83 | v55.2,105.78 54.7,106.28 LED1.P1-ANODE | v57,103.68 60.3,103.68 61.8,101.88 61.8,97.43 63,96.18 63,94.48 63.4,94.08 | 82.45,91.33 79.1,94.68 79,94.68 78.7,94.38 76.55,94.38 75.45,93.28 71.8,93.28 70.6,94.48 69.85,94.48 69.45,94.88 65,94.88 64.2,94.08 63.4,94.08 | 82.45,91.33 83.7,90.08 83.7,89.98 83.3,89.58 83.3,87.68 84.9,86.08 87.1,86.08 88.1,87.08 v88.15,86.88 | v51.1,51.83 51.1,47.38 v52.2,46.48 | v59.4,40.78 67,40.78 v68.3,39.48 | v77.8,35.88 77.7,35.78 v73.6,35.78 73.6,34.48 77.2,30.88 77.2,30.78 v77,30.58 | v89.9,31.28 90,31.28 90.55,30.73 | U$5.P$13 81.75,90.63 82.1,90.98 82.45,91.33 | U$7.P$1 76.5,79.41 76.5,78.88 | v90.2,88.38 90.2,89.2 LED2.P1-ANODE
  Top 0.2: 77.25,8.49 R8.1 | v74.4,30.08 72.99,30.08 U1.24 | U$5.P$4 80.15,88.53 80.3,88.68 80.3,89.53 | 80.3,89.53 80.3,89.98 80.4,90.08 81.5,90.08 81.7,90.28 81.7,90.58 | 80.3,89.53 U$5.P$2 | RA2.1B RA2.2B RA2.3B RA2.4B v16.7,33.48 16.5,33.38 16.5,29.63 16.35,29.48 16.35,29.08 16.05,28.78 12.35,28.78 12.3,28.73 9.95,28.73 9.65,28.43 9.65,26.33 9.62,26.3 U6.3 | v16.4,39.88 16.4,38.31 VR_IR.4 | R15.2 52.65,98.83 RA3.1B | 31.95,8.83 38.25,6.73 42.95,6.73 42.95,8.73 43.9,10.58 | 63.4,94.08 62.8,94.08 v62.15,93.63 | ADC2.2 12.21,63.24 v12.25,63.28 | LED3.P1-ANODE 96.4,61.13 v96.4,59.88 96.4,51.03 v95.8,50.43 | EEPROM.4 v63.04,81.49
  Top 0.254: RA3.1B RA3.2B RA3.3B RA3.4B RA1.1B RA1.2B RA1.3B RA1.4B | v20.3,44.78 C8.1 | 14.7,71.28 14.93,71.25 R3.1 R3.2 R3.3 R3.4 17.33,71.08 17.33,69.75 R5.1 R5.2 R5.3 R5.4 | 14.7,71.28 14.7,73.38 14.8,73.48 14.8,74.53 ADC1.6 | ADC1.6 ADC1.5 14.17,75.91 13.9,76.18 12.5,76.18 12.2,75.88 12.2,74.57 ADC1.2 | ADC1.6 14.83,76.31 16.4,77.88 17.3,77.88 18.7,79.28 18.7,81.18 18.9,81.38 18.9,82.48 18.9,82.88 18,83.78 17.4,83.78 R4.5 R4.6 R4.7 R4.8 | C3.1 13.8,70.53 | 13.8,70.53 13.95,70.53 14.7,71.28 | ADC2.15 14.83,67.85 14,68.68 14,69.23 14,70.33 13.8,70.53 | ADC2.6 ADC2.5 14.17,62.51 14,62.68 12.4,62.68 12.2,62.48 12.2,61.37 ADC2.2 | v93.3,38.08 93.3,37.98 92.5,36.98 92.5,32.68 90.55,30.73 90.3,30.48 90.3,29.88 91.6,28.58 93.3,28.58 v95.3,26.58 | LED6.P1-ANODE 12.6,17.68 v8.4,22.78 | v8.4,25.48 U6.3 | U$5.P$4 78.75,88.53 76.3,86.08 76.3,80.73 76.5,80.53 76.5,78.88 76.5,73.28 77.3,72.48 R24.2 77.35,71.68 78.3,71.68 78.45,71.53 78.45,65.43 79.25,64.63 U$20.1-VDD | 81.7,90.58 82.1,90.98 | v61.45,73.93 61.45,73.43 61.75,73.13
  Top 0.256: RA3.4B 51.29,102.69 50.5,103.48 50.5,104.03 49.95,104.58 48.85,104.58 48.65,104.78 48.65,107.23 48.8,107.38 52.15,107.38 LED1.P1-ANODE | LED4.P1-ANODE 87.05,15.93 v86,14.88 | 14,62.68 14,64.73 14.85,65.58 14.85,66.98 ADC2.15 | LED8.P1-ANODE 16.8,91.18 13.7,87.93 13.5,87.88 13.05,87.88 12.85,87.98 12.45,88.38 12.1,87.98 9.85,85.18 7.35,81.58 5.9,78.93 7.4,78.43 7.5,78.33 7.65,78.08 7.8,77.78 7.8,77.43 5.8,72.48 6.35,72.48 7.35,71.48 7.35,70.58 7.6,70.33 C4.1 v9.4,68.28 | v13.2,69.23 14,69.23 | U2.24 51.47,30.06 R2.2 52.65,29.18
  Top 0.305: 77.25,8.49 77.84,7.9
  Top 0.406: U$6.9-VDD 37.2,72.88 32.1,72.88 28.4,69.18 25.6,69.18 24.5,70.28 24.5,79.88 v23.7,80.68 | v21.7,82.68 19.1,82.68 18.9,82.48 | C14.2 43.35,11.13 43.9,10.58 45.6,10.58 46.8,9.38 49.72,9.38 U$3.4-VDD 50.91,10.79 51.2,11.08 51.2,12.18 v51.7,12.68 | v54,29.18 52.65,29.18
  Bottom 0.2: v50.8,68.48 49.8,68.48 49.1,69.18 40,69.18 v37.4,71.78 | v88.15,86.88 88.7,86.88 v90.2,88.38 95.4,82.18 97.4,78.18 96.1,77.68 96.7,76.28 97.05,75.38 97.05,71.93 96.75,71.63 96.4,71.63 | v57,103.68 v55.2,105.78 | v52.2,46.48 52.2,41.18 59,41.18 v59.4,40.78 | v68.3,39.48 68.3,39.28 70.5,37.08 70.9,37.08 71.6,36.38 73,36.38 v73.6,35.78 | v77.8,35.88 78.6,35.88 82.05,32.63 88.4,32.63 v89.9,31.28 | v77,30.58 76.6,30.18 74.5,30.18 v74.4,30.08 | v16.7,33.48 16.7,39.58 v16.4,39.88 | U$18.1-VDD 49.85,53.43 49.8,53.38 49.8,51.83 v51.1,51.83 51.3,52.03 57.95,52.03 58.2,52.28 58.2,54.78 57.9,55.08 U$26.VDD | v62.15,93.63 62.15,93.48 61.75,93.08 61.75,86.83 62.05,86.53 62.05,84.68 61.7,84.33 61.7,81.88 61.82,81.83 62.16,81.49 v63.04,81.49 | v96.4,59.88 96.4,71.63 | v12.25,63.28 12.25,62.78 11.1,61.63 U$25.P$1 | U$27.5 93.15,73.53 95.3,71.38 96.15,71.38 96.4,71.63
  Bottom 0.254: v20.3,44.78 20.3,40.88 18.6,40.88 17.75,40.03 16.55,40.03 v16.4,39.88 | v95.8,50.43 95.8,49.03 94.5,47.68 93.3,46.58 v93.3,38.08 | v95.3,26.58 95.2,25.98 94.8,25.18 90.9,19.58 v86,14.88 | v8.4,22.78 v8.4,25.48 | v63.04,81.49 63.04,77.17 61.75,75.88 61.75,74.23 v61.45,73.93
  Bottom 0.256: v9.4,68.28 13.2,68.33 v13.2,69.23
  Bottom 0.406: v23.7,80.68 v21.7,82.68 | v51.7,12.68 51.7,26.88 v54,29.18
V_MBED  (via drill 0.25 pad 0.6, 0.25 pad 0.65)
  Top 0.2: 65.6,84.78 v65.9,84.48 65.05,85.33 R13.2 62.7,84.18 59.95,84.18 59.8,84.33 | U4.1 67.93,85.21 67.95,85.23 | 59.8,84.33 57.15,84.33 56.85,84.03 R17.1 R16.1 56.35,80.73 56.35,80.28 | U$28.5V 56,70.53 56.35,70.88 56.35,80.28 | v51.7,81.48 51.75,81.48 v52.75,80.13 | v55.8,79.83 55.9,79.83 56.35,80.28 | R14.2 60.3,84.83 59.8,84.33
  Top 0.254: U$21.VCC-5V v10,40.08 | v23.3,59.43 25.3,61.43 25.3,66.38 v24.35,67.33 | v22.85,90.98 v24.65,90.98 | U$9.1-5V 43.2,92.48 43.5,92.18 46.4,92.18 46.5,92.08 46.5,86.28 | v90.85,67.48 94,70.28 94,76.23 92.85,77.38 90.9,77.38 90.2,78.08 90.2,79.68 91.35,80.83 R29.2
  Top 0.256: 46.5,86.28 46.5,86.13 v45.75,85.38
  Top 0.305: C19.1 74.02,86.06 | U$1.P$2 | 69.53,86.15 U4.15
  Top 0.42: C18.ANODE 81.17,68.35 v81.15,68.33
  Top 0.5: 71.9,87.03 71.85,87.03 71.75,86.93 69.75,86.93 69.6,86.78 69.6,86.12 U4.15 | 69.53,86.15 69,86.15 U4.16
  Top 0.6: 67.95,85.23 67.95,86.03 v67.65,86.33 67.88,86.1 U4.16 | 74.02,86.06 74.02,87.37 U$1.P$2 73.1,88.23 71.9,87.03 | v66.85,75.08 v70,75.08
  Bottom 0.2: 73.2,88.19 U$1.P$2 | U$22.VCC-5V 96.1,48.43 96.45,48.78 96.45,50.83 95.1,52.23 82.25,52.23 77.8,56.53 77.8,58.13 78.15,58.48 78.15,60.28 77.8,60.63 77.8,68.18 77.65,68.33 | 66,84.38 v65.9,84.48 | v52.75,80.13 52.75,79.98 52.95,79.73 55.7,79.73 v55.8,79.83
  Bottom 0.254: v10,40.08 10.3,40.38 10.3,41.18 10.35,52.43 11.25,53.28 17.2,53.33 v23.3,59.43 | v24.35,67.33 24.35,69.68 23.25,70.78 23.25,77.03 20.7,79.58 20.7,90.68 21,90.98 v22.85,90.98 | v24.65,90.98 25.45,90.98 26.6,92.13 32.3,92.13 33.55,93.38 U$9.1-5V | v90.85,67.48 90.85,66.88 89.7,65.73 87.35,65.73 85.7,67.38 82.1,67.38 v81.15,68.33
  Bottom 0.256: v45.75,85.38 45.75,83.88 47.65,81.98 51.2,81.98 v51.7,81.48
  Bottom 0.305: v67.65,86.33 67.65,86.23
  Bottom 0.406: U$1.P$42 U$1.P$2 | 69.95,75.03 v70,75.08
  Bottom 0.6: v66.85,75.08 65.75,76.18 65.75,84.33 v65.9,84.48 65.9,84.58 v67.65,86.33 | 69.95,75.03 70,75.03 70.05,74.98 70.05,73.03 70,72.98 70,72.93 69.95,72.88 69.95,71.58 71.05,70.48 75.5,70.48 77.65,68.33 | 77.8,68.18 78.25,68.63 80.85,68.63 v81.15,68.33
V_RECT  (via drill 0.35 pad 0.7)
  Top 0.305: U$11.P$2 26.45,25.73 v26.2,25.48 | v21.9,25.18 22.1,25.18 22.5,24.78 22.5,23.93 U$4.1 22.5,22.48 23.1,21.88 23.1,20.48 24.2,19.38 C16.1
  Top 0.406: U$17.4 15.15,19.23 17.2,17.18 19,17.18 19.15,17.03 23.7,17.03 23.9,16.83 24.9,16.83 25.4,17.33 25.4,18.78 C16.1
  Bottom 0.305: v26.2,25.48 26.2,26.18 24.7,26.18 24.1,25.58 22.6,25.58 v21.9,25.18
V_USB  (via drill 0.35 pad 0.7)
  Top 0.305: USB_CHARGE.2 71,67.88 71.9,66.98 71.9,61.98 73.1,60.78 73.1,52.78 72.7,52.38 v70.5,52.38 | v65.2,38.18 64.9,37.88 45.5,37.88 44.3,39.08 42.3,39.08 41.2,37.98 v40.4,37.98 | v29.1,28.78 29.1,27.38 28.3,26.58 27.8,26.58 U$11.P$1 | C17.1 24.1,21.68 23,22.93 U$4.2 22.99,24.77 23,25.28 v21.9,26.18
  Bottom 0.305: v70.5,52.38 65.6,52.38 64.7,51.48 64.7,43.08 65,42.78 65,38.08 v65.2,38.18 | v40.4,37.98 40.4,30.88 36.3,30.88 34.9,29.48 29.9,29.58 v29.1,28.78 25.2,26.88 24.2,26.88 24.2,26.48 23.9,26.18 v21.9,26.18
VIN  (via drill 0.25 pad 0.6, 0.25 pad 0.65, 0.35 pad 0.75)
  Top 0.2: C5.1 44.3,59.68 | v41,52.58 41.03,52.58 41.03,52.45 40.9,52.58 | PIC.5 52.6,6.68 52.6,5.78 51.5,4.68 50.1,4.68 49.4,3.98 46.6,3.98 U$19.5
  Top 0.254: VR_R.2 59.4,50.88 v59.4,53.38 | VR_L.2 41.03,52.45 | v12.7,28.18 12.7,27.69 12.71,27.68 | 13.44,24.27 13.44,21.91 v13.45,21.83 | v20.6,16.28 24.9,16.28 25.2,15.98 v31.7,15.98 | v34.25,16.08 35.25,16.08 v35.9,15.38 | v41.25,10.63 41.4,10.53 v41.4,7.43 | 13.83,36.76 v13.8,36.73 | v21.15,41.13 21.15,41.03 | 20.2,40.08 20.2,39.68 C9.1
  Top 0.305: 70.8,80.26 C20.2 | 70.94,82.07 U4.8
  Top 0.406: R25.2 13.44,24.27 13.44,27.13 13.26,27.3 13.26,27.31 12.89,27.68 12.89,27.69 12.71,27.68 12.44,27.68 | 13.83,36.76 VR_IR.2
  Top 0.42: C7.1 v58.1,59.68
  Top 0.5: 70.8,80.26 70.8,72.58 | 70.8,72.58 69.55,71.33 69.55,67.88 68.45,66.78 v62.55,66.78 | C20.2 70.94,82.07 | 70.8,72.58 v70.8,72.03 | v44.55,57.38 44.55,59.28 C5.1 44.2,59.68 44.95,60.43 56.95,60.43 v58.1,59.68 | U6.5 12.03,26.96 12.1,27.03 12.44,27.68
  Top 0.6: 40.9,52.58 39.35,52.58 38.85,52.08 38.85,46.43 38.25,45.83 30.25,45.83 29.15,44.73 21.55,44.73 v21.45,44.83 | 21.15,41.03 20.2,40.08 | v16,36.73 18.35,36.73 18.6,36.98 18.6,39.08 19.1,39.58 C9.1
  Top 0.813: v89.5,67.08 89.5,67 L2.2
  Bottom 0.254: v59.4,53.38 59.4,59.68 v58.1,59.68 | v31.7,15.98 32.75,15.98 32.85,16.08 v34.25,16.08 | v35.9,15.38 35.9,15.28 36.2,14.98 36.2,11.38 36.95,10.63 v41.25,10.63 | v41.4,7.43 41.4,5.58 41.6,5.38 40.9,2.98 44.2,2.28 U$19.5 | v13.45,21.83 13.6,21.83 13.7,21.78 14.9,20.43 14.9,19.68 17.75,16.83 20.05,16.83 v20.6,16.28
  Bottom 0.42: 59.3,66.78 59.3,66.63 59.2,66.53 59.2,60.33 58.55,59.68 v58.1,59.68
  Bottom 0.5: v62.55,66.78 59.3,66.78
  Bottom 0.6: v44.55,57.38 44.5,57.38 41,53.88 v41,52.58 | v21.15,41.13 21.15,44.53 v21.45,44.83 | v16,36.73 v13.8,36.73 13.8,32.13 13.1,31.43 11.75,31.43 10.8,30.48 10.8,28.98 11.2,28.58 12.7,28.58 v12.7,28.18
  Bottom 0.61: v70.8,72.03 82.3,72.03 84.3,70.03 85.9,68.38 v89.5,67.08
VOUT_MBED  (via drill 0.25 pad 0.65)
  Top 0.2: v79.6,60.33 77.65,60.33 v76.6,59.28 | U$23.8 87.98,63.09 88.2,62.88 88.2,60.63 87.95,60.38 v82.25,60.38
  Bottom 0.2: v82.25,60.38 79.65,60.38 v79.6,60.33 | v76.6,59.28 76.6,61.93 U$1.P$80
  Bottom 0.254: U$1.P$80 75.7,66.48 75.2,66.98 68,67.08 66.38,68.7 64.22,68.7 63.58,68.06 51.9,68.08 51.5,68.48 51.5,78.92 U$10.VCC
  Bottom 0.406: U$1.P$40 U$1.P$80
VPP2
  Top 0.2: U$7.P$4 81.31,77.72 81.9,77.13 82.95,77.13 83.3,76.78 85.9,76.78 86.25,76.43 90.85,76.43 91.15,76.13 U$27.4
VR_ENABLE  (via drill 0.25 pad 0.6, 0.25 pad 0.65)
  Top 0.2: VR_L.1 39.76,44.64 39.48,44.35 | 39.48,44.35 39.3,44.18 38.7,44.18 38.2,44.68 30.9,44.68 29.6,43.38 19.65,43.38 v17.05,40.78 | v12.6,40.38 12.6,38.32 VR_IR.1 | v42.6,9.33 42.6,10.73 42.35,10.98 42.35,12.28 v41.8,12.83 | v40.2,43.58 40.2,43.63 | v61.45,72.08 61.45,71.48 61.65,71.28 61.65,68.33 60.55,67.23 54.75,67.23 54.15,66.63 54.15,64.18 v54.1,64.13 | v52.05,59.63 52.3,59.88 56.75,59.88 57.35,59.28 57.35,57.98 58.16,57.22 VR_R.1 58.15,49.88 58.35,49.83 58.55,49.58 58.65,49.33 58.65,44.08 57.8,43.23 40.55,43.23 v40.2,43.58 | 39.48,44.35 39.48,44.3 v40.2,43.58 | v72.45,86.18 72.8,85.83 72.8,84.78 72.5,84.48 71.92,84.48 U4.11
  Top 0.256: PIC.4 51.66,5.74 v51.95,6.03
  Bottom 0.2: v17.05,40.78 13,40.78 v12.6,40.38 | v51.95,6.03 44.1,6.03 42.75,7.38 42.75,9.18 v42.6,9.33 | v41.8,12.83 41.8,37.03 41.25,37.58 41.25,42.53 v40.2,43.58 | v61.45,72.08 61.9,72.08 62.45,72.63 62.45,74.98 63.25,75.78 64.7,75.78 66.4,74.08 67.1,74.08 67.65,74.63 67.65,75.88 67.35,76.18 67.35,79.63 67.9,80.18 74.7,80.18 74.85,80.33 74.85,83.78 v72.45,86.18 | v54.1,64.13 54.05,61.33 v52.05,59.63
VSENSE  (via drill 0.25 pad 0.65, 0.25 pad 0.7, 0.4 pad 0.75, 0.4 pad 0.85)
  Top 0.2: U6.4 10.8,26.18
  Top 0.254: U$15.7 18.79,27.09 | 18.79,27.09 U$15.6 | 18.79,27.09 18.19,27.09 v17.91,26.71
  Top 0.406: U$15.4 18.62,28.29 v17.91,29.11 | v15.67,23.73 R25.1 | POWER.2 11.28,36.45 12.85,34.88 17,34.88 17.8,34.08 17.8,32.73 v17.3,32.23
  Top 0.6: 10.8,26.18 12.45,26.18 v12.63,26
  Bottom 0.6: v12.63,26 13.41,26 v15.67,23.73 17.91,25.97 v17.91,26.71 v17.91,29.11 17.2,29.81 17.2,32.03 17.3,32.13 v17.3,32.23

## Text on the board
Top: Psi-Swarm
Bottom: JAH 2015
tPlace: York Robotics Laboratory | PCB Version 1.5 | (C) J Hilder, Oct 2015
bPlace: C:/Users/James/Desktop/psi-swarm.bmp | PCB Version 1.5 / J. Hilder - Oct 2015
tNames: DC | CG | FULL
